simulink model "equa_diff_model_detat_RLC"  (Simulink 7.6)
settings: Solver=ode23tb  StartTime=0.0  StopTime=0.5  RelTol=1e-3
InitFcn:
  | close all
  | clc
  | clear all
  | % valeurs de R, L et C
  | R=3.3;
  | L=100e-3;
  | C=1e-3;

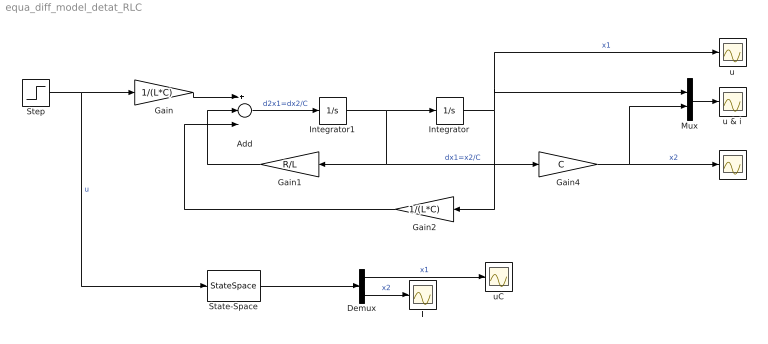
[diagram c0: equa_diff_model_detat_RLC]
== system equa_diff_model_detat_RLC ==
  Add : Sum  Inputs=+--
  Demux : Demux  Outputs=2
  Gain : Gain  Gain=1/(L*C)
  Gain1 : Gain  Gain=R/L
  Gain2 : Gain  Gain=1/(L*C)
  Gain4 : Gain  Gain=C
  Integrator : Integrator
  Integrator1 : Integrator  InitialCondition=0.01
  Mux : Mux  Inputs=2
  State-Space : StateSpace  A=[0 1/C;-1/L -R/L]  B=[0 1/L]'  C=[1 0;0 1]  D=[0 0]'  X0=[0 0.01]'
  Step : Step  Time=0.05  SampleTime=0
  i : Scope
  iL : Scope
  u : Scope
  u & i : Scope
  uC : Scope
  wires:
  Mux/1 -> u & i/1
  Integrator1/1 -> Integrator/1, Gain1/1, Gain4/1  "dx1=x2/C"
  Step/1 -> Gain/1, State-Space/1  "u"
  Gain/1 -> Add/1
  Integrator/1 -> Gain2/1, u/1, Mux/1  "x1"
  Gain1/1 -> Add/2
  Gain2/1 -> Add/3
  Add/1 -> Integrator1/1  "d2x1=dx2/C"
  Gain4/1 -> i/1, Mux/2  "x2"
  State-Space/1 -> Demux/1
  Demux/2 -> iL/1  "x2"
  Demux/1 -> uC/1  "x1"
